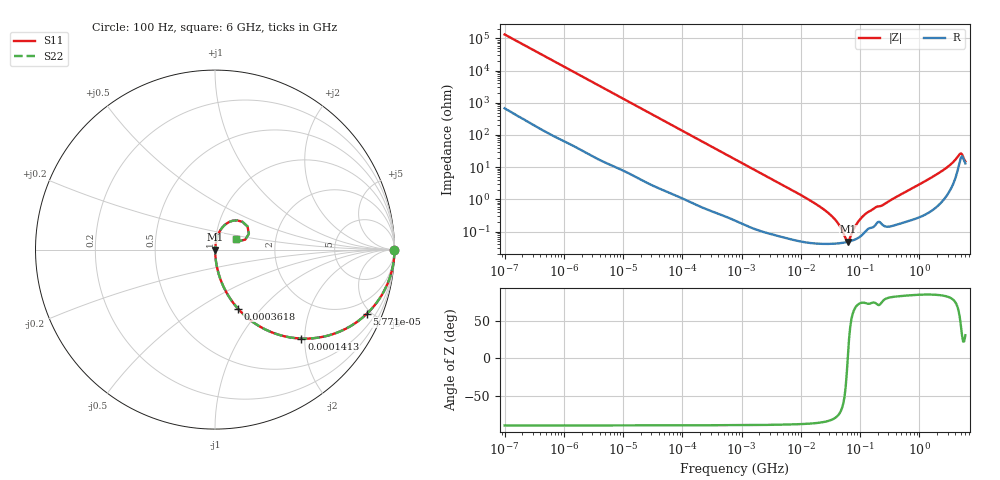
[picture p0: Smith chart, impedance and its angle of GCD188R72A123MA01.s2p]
!Murata Part Number: GCD188R72A123MA01
!These Parameters are Measured in Series Mode Connection
!Data Generated on Mar 13, 2026
!  o--ll--o
!Port1  Port2
!  o------o
!Operation Temp=25[degC], DC Bias Voltage=0[V]
!Freq. Start=100[Hz] Stop=6[GHz] 401[Steps]
# Hz S RI R 50
!Freq.(Hz) S11(Real) S11(Imag) S21(Real) S21(Imag) S12(Real) S12(Imag) S22(Real) S22(Imag)
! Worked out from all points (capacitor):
!   401 points, 100 Hz to 6 GHz, reference 50 ohm
!   read as one part in series: C = 12 nF near 109 Hz
!   lowest |Z| = 48 mohm at 62.33 MHz (marker M1)
!   series resonance near 61.96 MHz, so ESL is about 550 pH
!   S11 on the Smith chart (normalised r, x): 100 Hz: open; 57.71 kHz: 1.03, -4.70; 141.3 kHz: 1.02, -1.93; 361.8 kHz: 1.01, -0.76; 6 GHz: 1.26, +0.15
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100  1 -0.000753  4.4e-06 0.000753  4.4e-06 0.000753  1 -0.000753
2008  0.9997 -0.015  0.000299 0.015  0.000299 0.015  0.9997 -0.015
12041  0.9916 -0.0885  0.00843 0.0885  0.00843 0.0885  0.9916 -0.0885
40335  0.9171 -0.2726  0.0829 0.2726  0.0829 0.2726  0.9171 -0.2726
57709  0.845 -0.3584  0.155 0.3584  0.155 0.3584  0.845 -0.3584
141303  0.4819 -0.4956  0.5181 0.4956  0.5181 0.4956  0.4819 -0.4956
361830  0.1277 -0.3287  0.8723 0.3287  0.8723 0.3287  0.1277 -0.3287
774597  0.0326 -0.1715  0.9674 0.1715  0.9674 0.1715  0.0326 -0.1715
2481164  0.00404 -0.0555  0.996 0.0555  0.996 0.0555  0.00404 -0.0555
1.555665e7  0.000506 -0.00845  0.9995 0.00845  0.9995 0.00845  0.000506 -0.00845
3.64232e7  0.000426 -0.00253  0.9996 0.00253  0.9996 0.00253  0.000426 -0.00253
4.556224e7  0.000437 -0.00142  0.9996 0.00142  0.9996 0.00142  0.000437 -0.00142
5.699437e7  0.000463 -0.000381  0.9995 0.000381  0.9995 0.000381  0.000463 -0.000381
6.233367e7  0.000479 2.76e-05  0.9995 -2.76e-05  0.9995 -2.76e-05  0.000479 2.76e-05
8.918374e7  0.000611 0.00171  0.9994 -0.00171  0.9994 -0.00171  0.000611 0.00171
1.166697e8  0.000905 0.0031  0.9991 -0.0031  0.9991 -0.0031  0.000905 0.0031
3.124326e8  0.00151 0.00881  0.9985 -0.00881  0.9985 -0.00881  0.00151 0.00881
2.142435e9  0.0109 0.0646  0.9891 -0.0646  0.9891 -0.0646  0.0109 0.0646
3.505958e9  0.0378 0.1194  0.9622 -0.1194  0.9622 -0.1194  0.0378 0.1194
4.586474e9  0.1218 0.1629  0.8782 -0.1629  0.8782 -0.1629  0.1218 0.1629
5.016141e9  0.1811 0.129  0.8189 -0.129  0.8189 -0.129  0.1811 0.129
6e9  0.1195 0.0601  0.8805 -0.0601  0.8805 -0.0601  0.1195 0.0601
